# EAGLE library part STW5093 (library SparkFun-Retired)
STW5093 - PCM Audio Codec Never was a sparkfun component -- Stock available
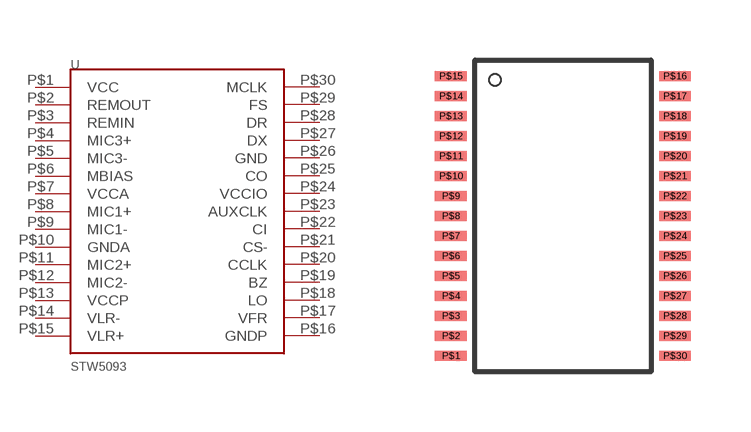
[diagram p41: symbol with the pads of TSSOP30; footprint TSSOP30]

Designator prefix -

## STW5093  [TSSOP30]
P$1  VCC
P$2  REMOUT
P$3  REMIN
P$4  MIC3+
P$5  MIC3-
P$6  MBIAS
P$7  VCCA
P$8  MIC1+
P$9  MIC1-
P$10  GNDA
P$11  MIC2+
P$12  MIC2-
P$13  VCCP
P$14  VLR-
P$15  VLR+
P$16  GNDP
P$17  VFR
P$18  LO
P$19  BZ
P$20  CCLK
P$21  CS-
P$22  CI
P$23  AUXCLK
P$24  VCCIO
P$25  CO
P$26  GND
P$27  DX
P$28  DR
P$29  FS
P$30  MCLK

## Footprint TSSOP30 (pad centres in mm)
smd 0.8 x 0.25: P$1 -2.8,-3.5; P$2 -2.8,-3; P$3 -2.8,-2.5; P$4 -2.8,-2; P$5 -2.8,-1.5; P$6 -2.8,-1; P$7 -2.8,-0.5; P$8 -2.8,0; P$9 -2.8,0.5; P$10 -2.8,1; P$11 -2.8,1.5; P$12 -2.8,2; P$13 -2.8,2.5; P$14 -2.8,3; P$15 -2.8,3.5; P$16 2.8,3.5; P$17 2.8,3; P$18 2.8,2.5; P$19 2.8,2; P$20 2.8,1.5; P$21 2.8,1; P$22 2.8,0.5; P$23 2.8,0; P$24 2.8,-0.5; P$25 2.8,-1; P$26 2.8,-1.5; P$27 2.8,-2; P$28 2.8,-2.5; P$29 2.8,-3; P$30 2.8,-3.5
